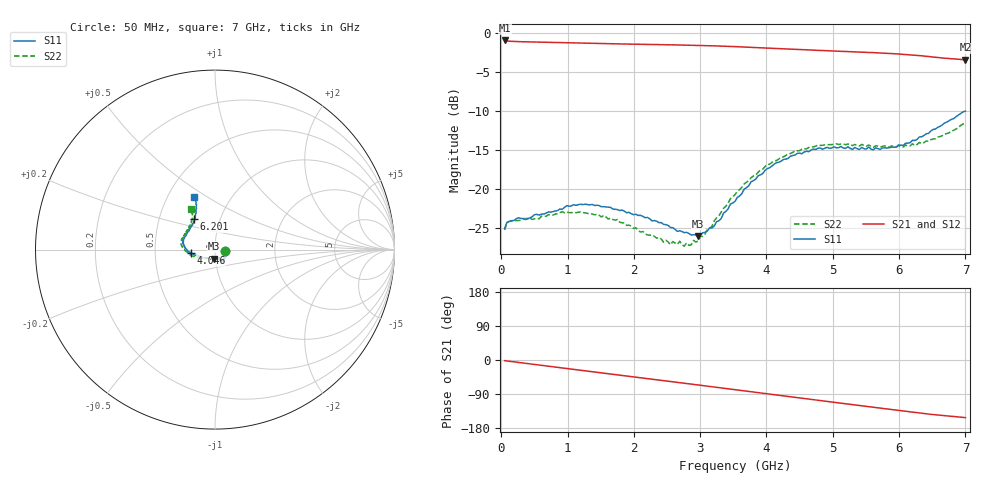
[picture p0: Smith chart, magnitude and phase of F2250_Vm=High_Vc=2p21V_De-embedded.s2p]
! Integrated Device Technology
! Corporate Headquarters
! 6024 Silver Creek Valley Road
! San Jose, CA 95138  USA
! Phone:  1-408-284-8200
! Toll Free:  1-800-223-1366
! Webpage:  http://www.idt.com/
! Timing and RF Division
! 515 Groton Road, Suite 102
! Westford, MA 01886-6024
! Device:  F2250
! Description: Voltage Variable RF Attenuator
! Frequency:  50.0 -  6000.00 MHz
! Package:  3x3 mm Thin QFN Plastic Package: 16 pin
! Ports:  2 RF, 3 DC
!  Pin  1  = GND
!  Pin  2  = NC
!  Pin  3  = RF1  = Port 1
!  Pin  4  = NC
!  Pin  5  = GND
!  Pin  6  = GND
!  Pin  7  = GND
!  Pin  8  = GND
!  Pin  9  = NC
!  Pin 10  = RF2  = Port 2
!  Pin 11  = NC
!  Pin 12  = GND
!  Pin 13  = GND
!  Pin 14  = VCNTRL
!  Pin 15  = VDD
!  Pin 16  = VMODE
! Vcntrl:  2.210 Volts
! Vmode:  +3.300 Volts
! Vdd:  +3.30  Volts
! Current:  1.316 mA
! Data:  The device was measured on a the F2250 evaluation board which has
!  individual transmission lines to the RF pins.  Data was collected
!  using a calibrated network analyzer.  The evaluation board was
!  de-embedded using a TRL calibration technique.
!  The reference plane is the edge of the package pin.
! Misc:  SN 10
!  Action Tracker AT0258
! Date Measured:  2014-11-26
! Date:  2015-10-15  MJV
! Note:
!  Integrated Device Technology supplies this data as a sample of measured
!  data at the package pin for this product.  Your particular data for this
!  product may vary.
!  Data was taken at 25 degrees C.
!  Integrated Device Technology reserves the right to change this data at anytime.
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# GHz S dB R 50
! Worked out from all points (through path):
!   201 points, 50 MHz to 7 GHz, reference 50 ohm
!   highest |S21| = -0.93 dB at 50 MHz (marker M1); lowest = -3.4 dB at 7 GHz (marker M2)
!   group delay of S21, straight-line fit = 61.1 ps
!   lowest |S11| = -26.0 dB at 2.969 GHz (marker M3), VSWR 1.11, Z = 49.4 - j4.94 ohm
!   |S11| at or under -10 dB: start of sweep to 6.999 GHz
!   |S22| runs from -27.3 to -11.5 dB; largest |S21 - S12| = 0.0019
!   S11 on the Smith chart (normalised r, x): 50 MHz: 1.12, -0.02; 4.046 GHz: 0.76, -0.03; 6.201 GHz: 0.75, +0.27; 7 GHz: 0.68, +0.44
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0.05  -25.07 -10.0  -0.93 -1.8  -0.93 -1.8  -25.25 -10.4
0.1195  -24.17 -9.7  -1.02 -3.2  -1.02 -3.2  -24.13 -8.6
0.57125  -23.33 -30.0  -1.14 -13.3  -1.14 -13.3  -23.81 -30.7
0.91875  -22.60 -48.2  -1.21 -21.0  -1.21 -21.1  -22.91 -49.9
1.2315  -21.99 -56.0  -1.28 -27.9  -1.28 -27.9  -23.02 -60.4
1.75275  -22.62 -62.9  -1.37 -39.1  -1.37 -39.1  -23.90 -67.2
2.37825  -24.31 -62.9  -1.46 -52.8  -1.46 -52.8  -26.21 -67.7
2.552  -24.93 -67.6  -1.48 -56.6  -1.48 -56.7  -27.14 -74.2
2.691  -25.35 -75.2  -1.51 -59.7  -1.51 -59.8  -26.70 -81.7
2.7605  -25.59 -77.3  -1.52 -61.3  -1.52 -61.3  -27.33 -86.1
2.969  -26.02 -94.3  -1.56 -66.0  -1.56 -66.0  -26.63 -104.7
3.21225  -24.73 -124.2  -1.62 -71.5  -1.62 -71.5  -24.07 -129.3
3.525  -21.59 -150.1  -1.72 -78.5  -1.72 -78.5  -20.72 -147.9
3.76825  -19.06 -162.8  -1.81 -84.0  -1.81 -84.0  -18.52 -159.0
4.04625  -17.27 -172.5  -1.92 -90.2  -1.92 -90.2  -16.81 -169.4
4.4285  -15.63 177.2  -2.07 -98.6  -2.07 -98.6  -15.10 179.1
4.7065  -14.86 170.2  -2.17 -104.8  -2.17 -104.8  -14.59 173.3
5.054  -14.71 162.0  -2.30 -112.5  -2.29 -112.5  -14.20 166.2
5.85325  -14.70 136.0  -2.59 -130.0  -2.59 -130.1  -14.60 147.4
6.20075  -13.74 124.3  -2.80 -137.7  -2.80 -137.8  -14.19 138.4
6.54825  -12.30 116.2  -3.07 -144.7  -3.08 -144.8  -13.53 127.0
7  -10.00 111.2  -3.40 -152.1  -3.41 -152.2  -11.52 120.8
